(* Logix 5000 DataType export Unit_Type; software revision 20.01 *)

TYPE Unit_Type :   // Common information for a unit
STRUCT
   Alm_Reset : BOOL;   // Alarm reset
   Local : BOOL;   // Local/remote control indication
   Maint : BOOL;   // Maintenance privilege for device control
   Man_StartOpen : BOOL;   // Manual start/open from operator
   Man_StopClose : BOOL;   // Manual stop/close from operator
   Man_DevNum : DINT;   // Number of device started/stopped at OI
   Msg : DINT;   // Message number
   Time_Remaining : DINT;   // Remaining time in timed steps
END_STRUCT
END_TYPE
